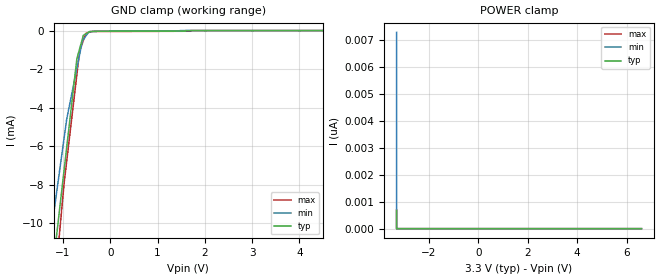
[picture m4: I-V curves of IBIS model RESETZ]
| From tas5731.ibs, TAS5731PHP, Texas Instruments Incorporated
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[Model]   RESETZ
Model_type   Input
Vinl = .8
Vinh = 2
|   typ   min   max
C_comp   0.7443p   0.7440p   0.7473p
[Voltage Range]   3.3   3   3.6
[Temperature Range]   27   125   0
[Power Clamp Reference]   3.3   3   3.6
[GND Clamp Reference]   -0   -0   -0
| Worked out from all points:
|   GND clamp passes 1 mA (typ) near -0.65 V on its own axis
[GND Clamp]
|   Voltage   I(typ)   I(min)   I(max)
-3.3V     -1.514A    -1.356A    -1.56A
-1.44V    -17.17mA   -13.87mA   -20.39mA
-978.5mV  -7.295mA   -5.624mA   -7.992mA
-922.7mV  -6.102mA   -4.627mA   -6.825mA
-706.1mV  -1.465mA   -1.966mA   -2.289mA
-648.4mV  -952.5uA   -1.257mA   -1.08mA
-590.9mV  -442.2uA   -551uA     -670.5uA
-568.4mV  -242.7uA   -472.3uA   -510.4uA
-516.3mV  -167.3uA   -289.9uA   -139.2uA
-430.7mV  -43.41uA   -71.21uA   -80.98uA
1.701V    0A         0A         0A
6.6V      0A         0A         0A
[POWER Clamp]
|   Voltage   I(typ)   I(min)   I(max)
-3.3V     677.8pA    7.274nA    698.9pA
-3.3V     0A         402pA      0A
-3.3V     0A         0A         0A
6.6V      0A         0A         0A
